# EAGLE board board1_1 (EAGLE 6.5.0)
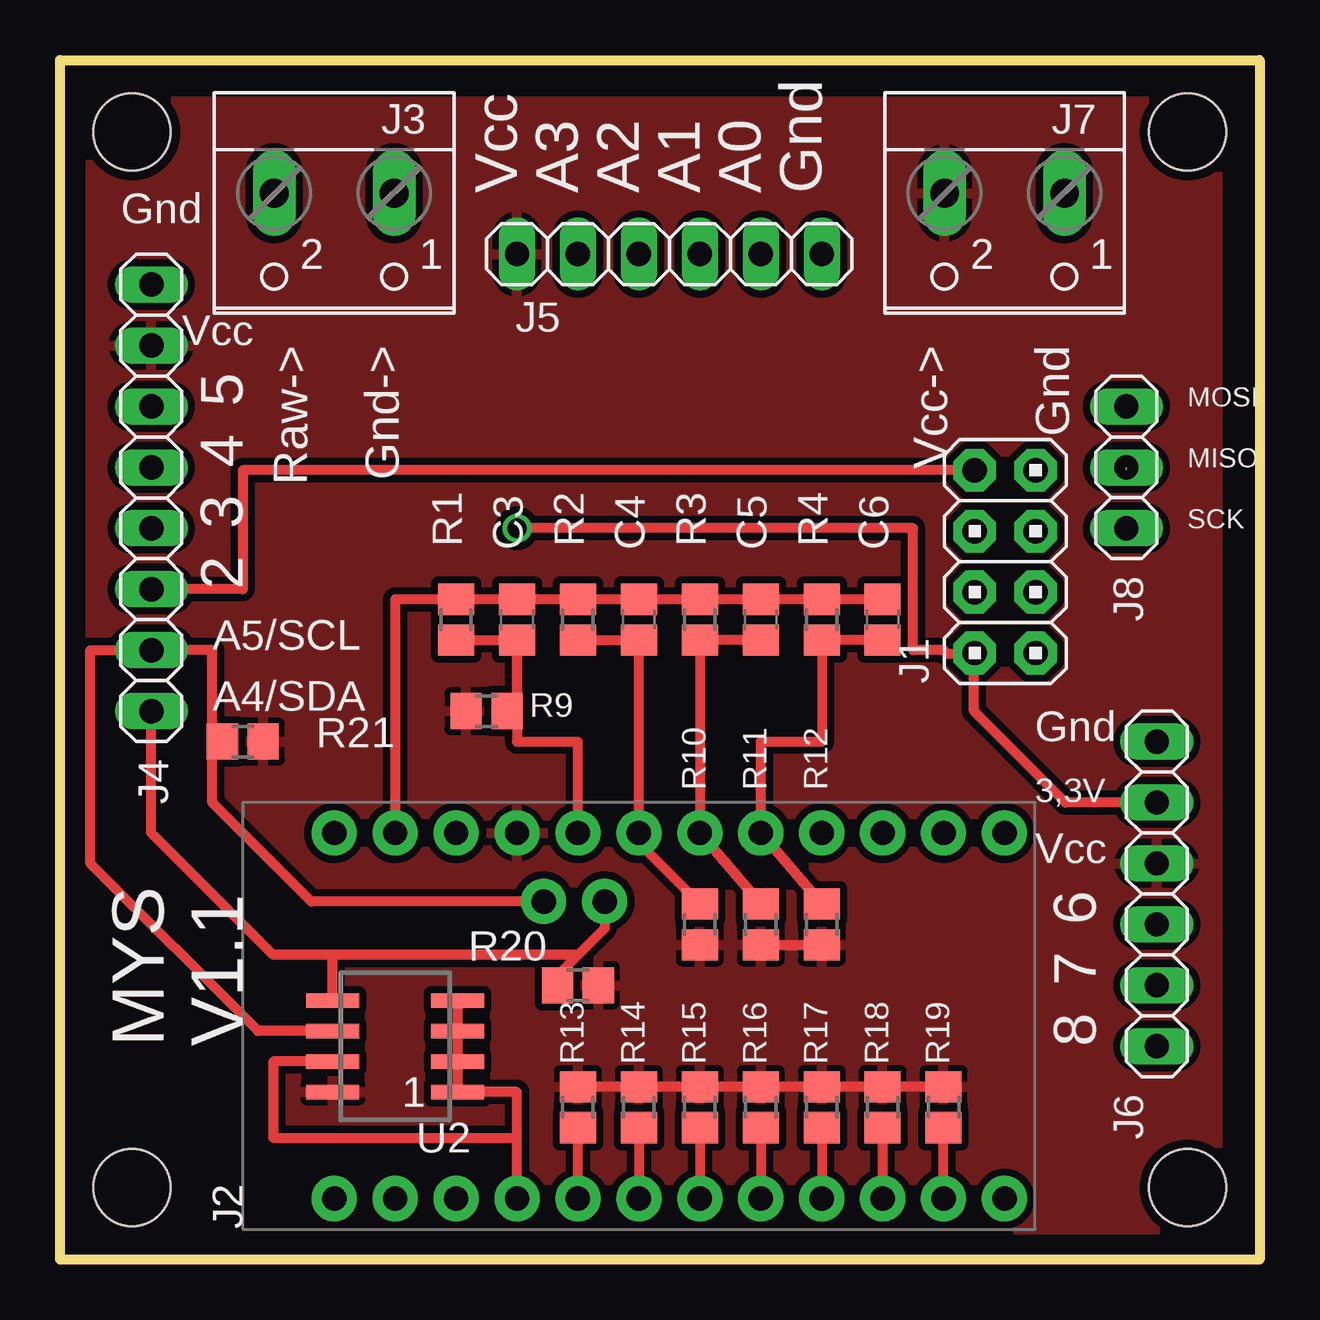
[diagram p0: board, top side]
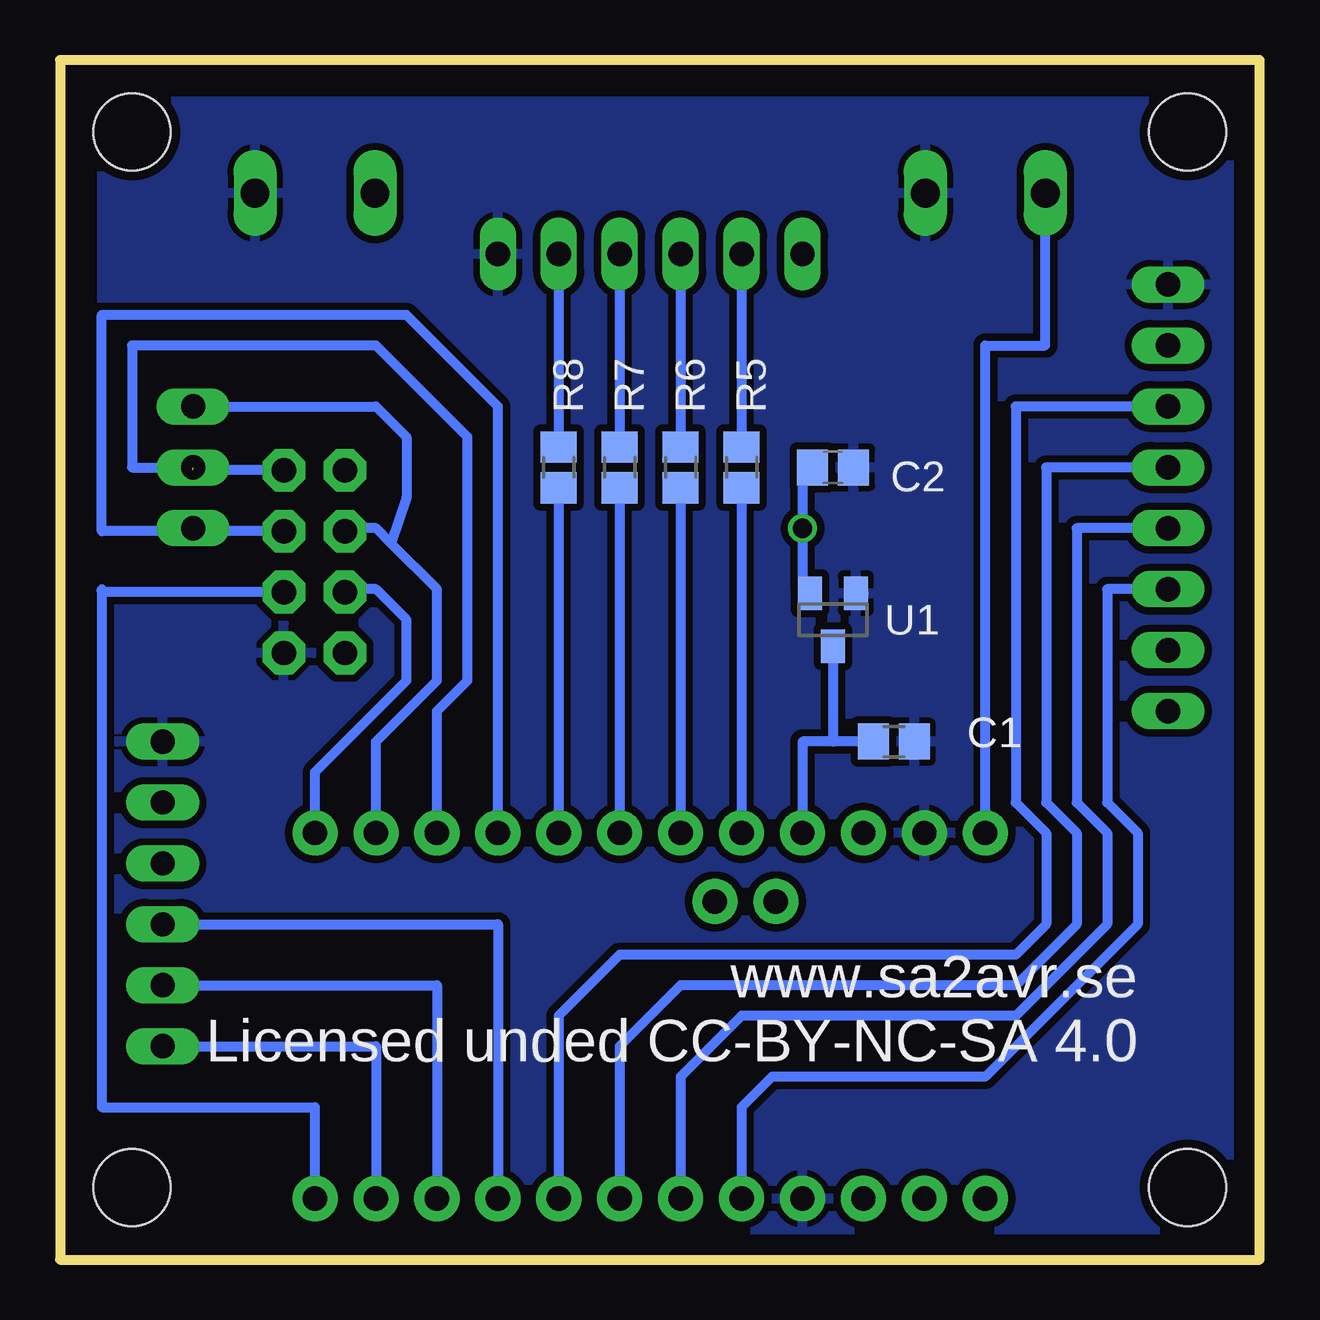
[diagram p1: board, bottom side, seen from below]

Size 50 x 50 mm. Coordinates in mm from the lower left corner, seen from the top.
Outline: 0,0 0,50 50,50 50,0 0,0
Copper layers (1*16): Top 0.035mm / dielectric 1.5mm / Bottom 0.035mm
Design rules "board": minimum track width 10mil, minimum drill 24mil, track to track 0.205mm, track to pad 0.205mm, pad to pad 0.205mm, via to via 0.205mm, smd to smd 8mil, copper to edge 0.4mm, drill to drill 0.25mm, minimum pad ring 10mil, minimum via ring 8mil, stop-mask expansion 4mil, vias tented up to drill 0mil, thermal gap 10mil
Holes 3.2 mm at 47,3 47,47 3,47 3,3

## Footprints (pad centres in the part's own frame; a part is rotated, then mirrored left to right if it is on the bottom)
R0805 = smd 1.3 x 1.5: 1 -0.85,0; 2 0.85,0
C0805 = smd 1.3 x 1.5: 1 -0.85,0; 2 0.85,0
2X04 = drill 1.016 pad 1.778 octagon: 1 -3.81,-1.27; 2 -3.81,1.27; 3 -1.27,-1.27; 4 -1.27,1.27; 5 1.27,-1.27; 6 1.27,1.27; 7 3.81,-1.27; 8 3.81,1.27
ARDUINO_PRO_MINI = drill 1.016 pad 1.88: 1 -7.62,12.7; 2 -7.62,10.16; 3 -7.62,7.62; 4 -7.62,5.08; 5 -7.62,2.54; 6 -7.62,0; 7 -7.62,-2.54; 8 -7.62,-5.08; 9 -7.62,-7.62; 10 -7.62,-10.16; 11 -7.62,-12.7; 12 -7.62,-15.24; 13 7.62,-15.24; 14 7.62,-12.7; 15 7.62,-10.16; 16 7.62,-7.62; 17 7.62,-5.08; 18 7.62,-2.54; 19 7.62,0; 20 7.62,2.54; 21 7.62,5.08; 22 7.62,7.62; 23 7.62,10.16; 24 7.62,12.7; A4 4.763,1.429; A5 4.763,3.969
W237-102 = drill 1.194 long: 1 -2.5,-1.27; 2 2.5,-1.27
1X08 = drill 1.016 long: 1 -8.89,0; 2 -6.35,0; 3 -3.81,0; 4 -1.27,0; 5 1.27,0; 6 3.81,0; 7 6.35,0; 8 8.89,0
1X06 = drill 1.016 long: 1 -6.35,0; 2 -3.81,0; 3 -1.27,0; 4 1.27,0; 5 3.81,0; 6 6.35,0
1X03 = drill 1.016 long: 1 -2.54,0; 2 0,0; 3 2.54,0
SOT23 = smd 1 x 1.4: 1 -0.95,-1.1; 2 0.95,-1.1; 3 0,1.1
SOP08 = smd 0.6 x 2.2: 1 -1.905,-2.6; 2 -0.635,-2.6; 3 0.635,-2.6; 4 1.905,-2.6; 5 1.905,2.6; 6 0.635,2.6; 7 -0.635,2.6; 8 -1.905,2.6

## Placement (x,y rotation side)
C1  [R0805]  15.24,21.59 0 bottom
C2  [C0805]  17.78,33.02 180 bottom
C3  [C0805]  19.05,26.67 90 top
C4  [C0805]  24.13,26.67 90 top
C5  [C0805]  29.21,26.67 90 top
C6  [C0805]  34.29,26.67 90 top
J1  [2X04]  39.4,29.09 90 top
J2  [ARDUINO_PRO_MINI]  24.13,10.16 90 top
J3  [W237-102]  11.43,43.18 180 top
J4  [1X08]  3.81,31.75 90 top
J5  [1X06]  25.4,41.91 0 top
J6  [1X06]  45.72,15.24 90 top
J7  [W237-102]  39.37,43.18 180 top
J8  [1X03]  44.45,33.02 90 top
R1  [R0805]  16.51,26.67 90 top
R2  [R0805]  21.59,26.67 90 top
R3  [R0805]  26.67,26.67 90 top
R4  [R0805]  31.75,26.67 90 top
R5  [R0805]  21.59,33.02 270 bottom
R6  [R0805]  24.13,33.02 270 bottom
R7  [R0805]  26.67,33.02 270 bottom
R8  [R0805]  29.21,33.02 270 bottom
R9  [R0805]  17.78,22.86 0 top
R10  [R0805]  26.67,13.97 90 top
R11  [R0805]  29.21,13.97 90 top
R12  [R0805]  31.75,13.97 90 top
R13  [R0805]  21.59,6.35 90 top
R14  [R0805]  24.13,6.35 90 top
R15  [R0805]  26.67,6.35 90 top
R16  [R0805]  29.21,6.35 90 top
R17  [R0805]  31.75,6.35 90 top
R18  [R0805]  34.29,6.35 90 top
R19  [R0805]  36.83,6.35 90 top
R20  [R0805]  21.59,11.43 0 top
R21  [R0805]  7.62,21.59 0 top
U1  [SOT23]  17.78,26.67 180 bottom
U2  [SOP08]  13.97,8.89 90 top

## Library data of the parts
C1-C6 R1-R21 = resistor
J1 J4-J6 J8 = pinhead
J2 = SparkFun-Robert
J3 J7 = con-wago-500
U1 = v-reg
U2 = ref-packages

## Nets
GND: C1.2 C2.1 C3.2 C4.2 C5.2 C6.2 J1.1 J2.4 J2.23 J3.1 J4.8 J5.6 J6.6 J7.1 R1.2 R2.2 R3.2 R4.2 U1.1 U2.1 U2.2 U2.3 U2.4 U2.7
RAW: J2.24 J3.2
S$1: J1.3 J2.12
S$2: J1.4 J2.13
S$3: J1.5 J2.16 J8.1
S$4: J1.6 J2.14 J8.3
S$5: J1.8 J2.5 J4.3 R13.1
S$6: J1.7 J2.15 J8.2
S$7: C6.1 J2.17 R4.1 R8.2 R12.2
S$8: J5.2 R5.1
S$9: C2.2 J1.2 J6.5 U1.2
S$10: J2.A5 J4.2 R21.1 U2.6
S$11: C5.1 J2.18 R3.1 R7.2 R11.2
S$12: C4.1 J2.19 R2.1 R6.2 R10.2
S$13: C3.1 J2.20 R1.1 R5.2 R9.2
S$14: J2.6 J4.4 R14.1
S$15: J5.3 R6.1
S$16: J5.4 R7.1
S$17: J2.11 J6.1 R19.1
S$18: J2.10 J6.2 R18.1
S$19: J2.9 J6.3 R17.1
S$20: J5.5 R8.1
S$21: J2.7 J4.5 R15.1
S$22: J2.8 J4.6 R16.1
S$23: J2.A4 J4.1 R20.1 U2.5
VCC: C1.1 J2.21 J4.7 J5.1 J6.4 J7.2 R9.1 R10.1 R11.1 R12.1 R13.2 R14.2 R15.2 R16.2 R17.2 R18.2 R19.2 R20.2 R21.2 U1.3 U2.8

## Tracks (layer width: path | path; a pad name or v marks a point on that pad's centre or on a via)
GND
  Top 0.406: C6.2 R4.2 C5.2 R3.2 C4.2 R2.2 C3.2 R1.2 13.97,27.52 J2.23 | U2.4 U2.3 U2.2 U2.1 19.05,6.99 19.05,5.08 | J2.4 19.05,5.08 | U2.7 8.89,8.26 8.89,5.08 19.05,5.08
  Bottom 0.406: U1.1 16.51,27.77
  pour Bottom (isolate 0.305, rank 3): 1.27,48.26 48.26,48.26 48.26,1.27 1.27,1.27
RAW
  Bottom 0.406: J3.2 8.93,38.1 11.43,38.1 J2.24
S$1
  Bottom 0.406: J1.3 48.26,27.82 | 48.26,27.82 48.26,27.94 | 48.26,27.82 48.26,6.35 39.37,6.35 J2.12
S$2
  Bottom 0.406: J2.13 39.37,20.32 35.56,24.13 35.56,26.67 36.83,27.94 38.01,27.94 J1.4
S$3
  Bottom 0.406: J2.16 31.75,35.56 35.56,39.37 48.26,39.37 48.26,30.36 J1.5 44.33,30.36 J8.1
S$4
  Bottom 0.406: J2.14 36.83,21.59 34.29,24.13 34.29,27.94 36.2,29.84 | 36.2,29.84 36.83,30.48 38.01,30.48 J1.6 | J8.3 36.83,35.56 35.56,34.29 35.56,31.75 36.2,29.84
S$5
  Top 0.406: J1.8 7.62,32.9 7.62,27.94 J4.3 | J2.5 R13.1
  Bottom 0.406: J4.3 6.35,27.94 6.35,19.05 5.08,17.78 5.08,13.97 11.43,7.62 20.32,7.62 21.59,6.35 J2.5
S$6  (1 unrouted)
  Bottom 0.406: J1.7 44.45,32.9 | 44.45,32.9 45.72,32.9 | J2.15 34.29,22.86 33.02,24.13 33.02,34.29 36.83,38.1 46.99,38.1 46.99,33.02 44.57,33.02 44.45,32.9
S$7
  Top 0.406: C6.1 R4.1 31.75,21.59 29.21,21.59 J2.17 R12.2
  Bottom 0.406: R8.2 J2.17
S$8
  Bottom 0.406: J5.2 R5.1
S$9  (via drill 0.8)
  Top 0.406: J6.5 41.91,19.05 38.1,22.86 38.1,25.25 | 38.1,25.25 J1.2 | 38.1,25.25 36.98,25.25 36.83,25.4 35.56,25.4 35.56,30.48 v19.05,30.48
  Bottom 0.406: C2.2 19.05,33.02 v19.05,30.48 19.05,27.94 18.73,27.94 U1.2
S$10
  Top 0.406: J2.A5 10.48,14.92 6.35,19.05 6.35,21.59 | 6.35,21.59 6.35,25.4 J4.2 1.27,25.4 1.27,16.51 8.26,9.53 U2.6 | R21.1 6.35,21.59
S$11
  Top 0.406: C5.1 R3.1 | R3.1 26.13,25.82 | R11.2 J2.18 R3.1
  Bottom 0.406: R7.2 J2.18
S$12
  Top 0.406: R2.1 C4.1 | C4.1 23.59,25.82 | C4.1 J2.19 24.13,17.36 R10.2
  Bottom 0.406: R6.2 J2.19
S$13
  Top 0.406: R9.2 19.05,22.86 C3.1 | R1.1 C3.1 | C3.1 19.05,21.59 21.59,21.59 J2.20
  Bottom 0.406: R5.2 J2.20
S$14
  Top 0.406: R14.1 J2.6
  Bottom 0.406: J4.4 7.62,30.48 7.62,19.05 6.35,17.78 6.35,13.97 10.16,10.16 21.59,10.16 24.13,7.62 J2.6
S$15
  Bottom 0.406: J5.3 R6.1
S$16
  Bottom 0.406: J5.4 R7.1
S$17
  Top 0.406: J2.11 R19.1
  Bottom 0.406: J6.1 36.83,8.89 J2.11
S$18
  Top 0.406: R18.1 J2.10
  Bottom 0.406: J6.2 34.29,11.43 J2.10
S$19
  Top 0.406: R17.1 J2.9
  Bottom 0.406: J6.3 31.75,13.97 J2.9
S$20
  Bottom 0.406: J5.5 R8.1
S$21
  Top 0.406: R15.1 J2.7
  Bottom 0.406: J4.5 8.89,33.02 8.89,19.05 7.62,17.78 7.62,13.97 10.16,11.43 24.13,11.43 26.67,8.89 J2.7
S$22
  Top 0.406: R16.1 J2.8
  Bottom 0.406: J4.6 10.16,35.56 10.16,19.05 8.89,17.78 8.89,13.97 10.16,12.7 26.67,12.7 29.21,10.16 J2.8
S$23
  Top 0.406: J2.A4 22.7,13.81 21.59,12.7 | 21.59,12.7 11.43,12.7 | 11.43,12.7 8.89,12.7 3.81,17.78 J4.1 | U2.5 11.37,12.64 11.43,12.7 | R20.1 20.74,11.85 21.59,12.7
VCC
  Top 0.406: R11.1 R12.1 | R19.2 R18.2 R17.2 R16.2 R15.2 R14.2 R13.2
  Bottom 0.406: 17.78,21.59 19.05,21.59 J2.21 | C1.1 17.78,21.59 | U1.3 17.78,21.59
  pour Top (isolate 0.305, rank 3): 1.27,48.26 1.27,1.27 48.26,1.27 48.26,48.26

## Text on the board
tNames: Vcc | A3 | A2 | A1 | A0 | Gnd | Gnd | Vcc | Raw-> | Gnd-> | Vcc-> | Gnd | 5 | MOSI | 4 | MISO | 3 | SCK | 2 | A5/SCL | A4/SDA | Gnd | 3,3V | Vcc | 6 | 7 | MYS / V1.1 | 8
bNames: www.sa2avr.se / Licensed unded CC-BY-NC-SA 4.0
